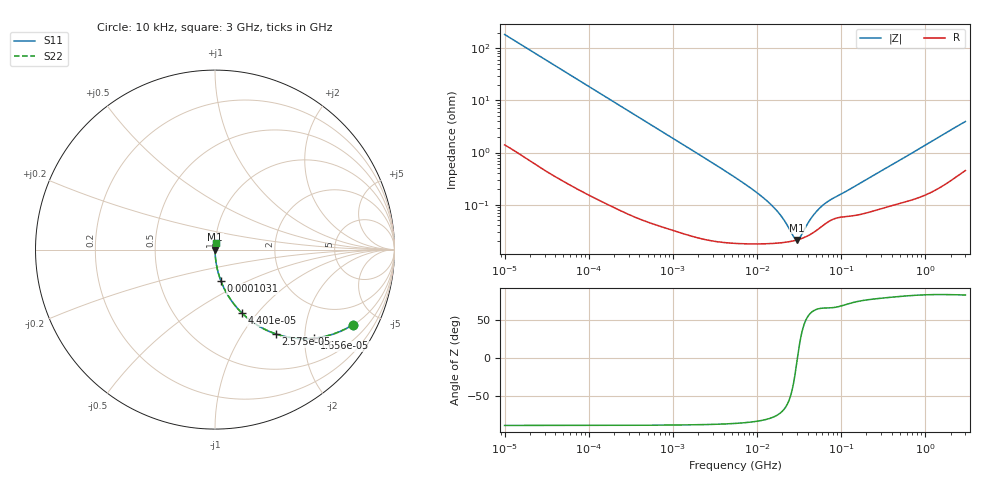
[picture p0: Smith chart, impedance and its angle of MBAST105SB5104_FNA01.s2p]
! MBAST105SB5104_FNA01  S-PARAMETER MODEL  ( Standard Model )
! Model Generated by TAIYO YUDEN Corporation (http://www.ty-top.com)
! Version 1.0
! TAIYO YUDEN Control No. 220601
! Copyright(c) 2013 TAIYO YUDEN CO.,LTD. All Rights Reserved.
! Product Description (link to TY-COMPAS)
! https://ds.yuden.co.jp/TYCOMPAS/or/detail?pn=MBAST105SB5104KFNA01&u=M
! Products Name : Multilayer Ceramic Capacitors
! Characteristics :
!  Capacitance : 0.1 [uF] , Rated Voltage : 25 [V] , TCC : X5R
!  Case Size : 1.0 x 0.5 / 0.039 x 0.02 [mm/inch] , Thickness : 0.5 / 0.02 [mm/inch]
!  (Conditions: Temperature = 25 [degC] , DC Bias Voltage = 0 [V])
! External Node Assignments :
!  1  o---| |---o  2
! GND o---------o GND
! Frequency Range : 10kHz  -  3GHz  [ 401 STEP ]
# MHZ S RI R 50
! Freq[MHz].  S11 Real  S11 Imag  S21 Real  S21 Imag  S12 Real  S12 Imag  S22 Real  S22 Imag
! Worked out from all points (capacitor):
!   401 points, 10 kHz to 3 GHz, reference 50 ohm
!   read as one part in series: C = 86.6 nF near 10.65 kHz
!   lowest |Z| = 21.1 mohm at 30.06 MHz (marker M1)
!   series resonance near 30.26 MHz, so ESL is about 320 pH
!   S11 on the Smith chart (normalised r, x): 10 kHz: 1.03, -3.67; 16.56 kHz: 1.02, -2.22; 25.75 kHz: 1.01, -1.43; 44.01 kHz: 1.01, -0.84; 103.1 kHz: 1.00, -0.36; 3 GHz: 1.01, +0.08
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0.01  0.7694 -0.4174  0.2306 0.4174  0.2306 0.4174  0.7694 -0.4174
0.016561  0.5523 -0.4935  0.4477 0.4935  0.4477 0.4935  0.5523 -0.4935
0.02575  0.3403 -0.4701  0.6597 0.4701  0.6597 0.4701  0.3403 -0.4701
0.034199  0.2275 -0.4155  0.7725 0.4155  0.7725 0.4155  0.2275 -0.4155
0.044011  0.1519 -0.3552  0.8481 0.3552  0.8481 0.3552  0.1519 -0.3552
0.082683  0.0494 -0.2128  0.9506 0.2128  0.9506 0.2128  0.0494 -0.2128
0.103102  0.0327 -0.1738  0.9673 0.1738  0.9673 0.1738  0.0327 -0.1738
0.234035  0.00706 -0.079  0.9929 0.079  0.9929 0.079  0.00706 -0.079
0.683653  0.00114 -0.0273  0.9989 0.0273  0.9989 0.0273  0.00114 -0.0273
5.477226  0.000192 -0.00334  0.9998 0.00334  0.9998 0.00334  0.000192 -0.00334
9.97066  0.00018 -0.00169  0.9998 0.00169  0.9998 0.00169  0.00018 -0.00169
15.02209  0.000181 -0.000951  0.9998 0.000951  0.9998 0.000951  0.000181 -0.000951
19.95104  0.000187 -0.000538  0.9998 0.000538  0.9998 0.000538  0.000187 -0.000538
27.34599  0.000203 -0.000127  0.9998 0.000127  0.9998 0.000127  0.000203 -0.000127
30.05882  0.000211 -8.44e-06  0.9998 8.44e-06  0.9998 8.44e-06  0.000211 -8.44e-06
33.04079  0.000221 0.00011  0.9998 -0.00011  0.9998 -0.00011  0.000221 0.00011
39.92153  0.000252 0.000351  0.9997 -0.000351  0.9997 -0.000351  0.000252 0.000351
45.28751  0.000282 0.000514  0.9997 -0.000514  0.9997 -0.000514  0.000282 0.000514
56.47134  0.000364 0.000801  0.9996 -0.000801  0.9996 -0.000801  0.000364 0.000801
70.41703  0.000471 0.00107  0.9995 -0.00107  0.9995 -0.00107  0.000471 0.00107
374.4521  0.000957 0.00538  0.999 -0.00538  0.999 -0.00538  0.000957 0.00538
3000  0.00601 0.0387  0.994 -0.0387  0.994 -0.0387  0.00601 0.0387
